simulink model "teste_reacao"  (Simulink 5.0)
settings: Solver=ode5  StartTime=0.0  StopTime=100  FixedStep=0.002  RelTol=1e-3
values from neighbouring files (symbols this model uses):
  CA0 = 12.815    [dados_19_2.m]
  CB0 = 0    [dados_19_2.m]
  k10 = 729.55    [dados_19_2.m]
  k20 = 6567.6    [dados_19_2.m]
  Lambda1 = 22222    [dados_19_2.m]
  Lambda2 = 27778    [dados_19_2.m]
  R = 1.9858    [dados_19_2.m]
  V = 1.2035    [dados_19_2.m]
libraries: simulink x1

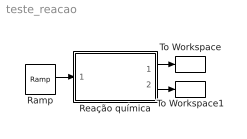
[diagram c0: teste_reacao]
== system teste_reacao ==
  Ramp : simulink/Sources/Ramp  slope=1  start=0  X0=25
  Reação química : Subsystem
  To Workspace : ToWorkspace  VariableName=q1  SampleTime=-1  SaveFormat=Array
  To Workspace1 : ToWorkspace  VariableName=q2  SampleTime=-1  SaveFormat=Array
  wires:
  Ramp/1 -> Reação química/1(T)
  Reação química/1(q1) -> To Workspace/1
  Reação química/2(q2) -> To Workspace1/1

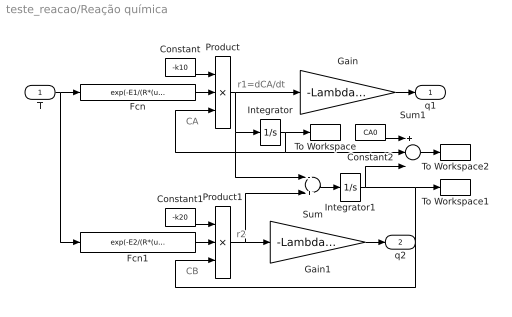
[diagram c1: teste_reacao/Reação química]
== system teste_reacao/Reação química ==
  note: CA
  note: r1=dCA/dt
  note: CB
  note: r2
  T : Inport
  Constant : Constant  Value=-k10
  Constant1 : Constant  Value=-k20
  Constant2 : Constant  Value=CA0
  Fcn : Fcn  Expr=exp(-E1/(R*(u+273.15)))
  Fcn1 : Fcn  Expr=exp(-E2/(R*(u+273.15)))
  Gain : Gain  Gain=-Lambda1*V
  Gain1 : Gain  Gain=-Lambda2*V
  Integrator : Integrator  InitialCondition=CA0
  Integrator1 : Integrator  InitialCondition=CB0
  Product : Product  Inputs=3
  Product1 : Product  Inputs=3
  Sum : Sum  Inputs=-+
  Sum1 : Sum  Inputs=+--
  To Workspace : ToWorkspace  VariableName=CA  SampleTime=-1  SaveFormat=Array
  To Workspace1 : ToWorkspace  VariableName=CB  SampleTime=-1  SaveFormat=Array
  To Workspace2 : ToWorkspace  VariableName=CC  SampleTime=-1  SaveFormat=Array
  q1 : Outport
  q2 : Outport  Port=2
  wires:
  T/1 -> Fcn/1, Fcn1/1
  Fcn/1 -> Product/2
  Constant/1 -> Product/1
  Product/1 -> Gain/1, Integrator/1, Sum/1
  Fcn1/1 -> Product1/2
  Product1/1 -> Gain1/1, Sum/2
  Gain/1 -> q1/1
  Gain1/1 -> q2/1
  Integrator/1 -> To Workspace/1, Sum1/2, Product/3
  Integrator1/1 -> Sum1/3, To Workspace1/1, Product1/3
  Sum/1 -> Integrator1/1
  Constant2/1 -> Sum1/1
  Sum1/1 -> To Workspace2/1
  Constant1/1 -> Product1/1
